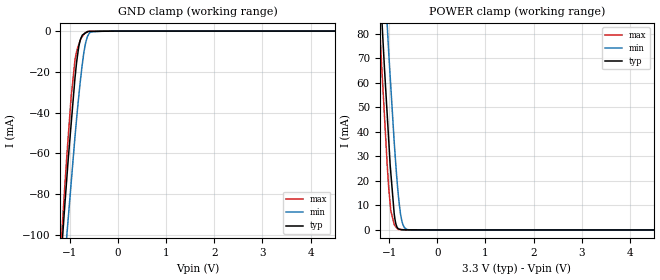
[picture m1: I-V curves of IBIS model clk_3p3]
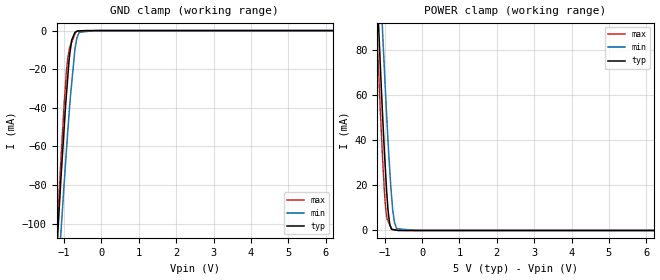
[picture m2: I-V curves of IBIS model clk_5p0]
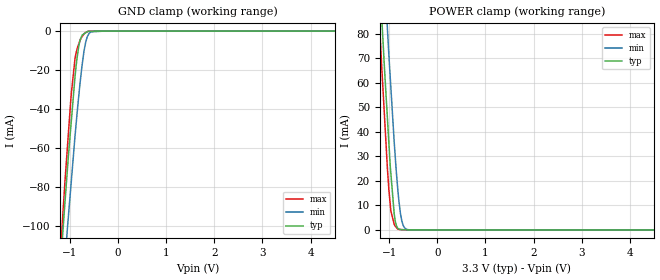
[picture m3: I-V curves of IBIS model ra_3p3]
|Texas Instruments Incorporated
| 10-Bit, 6 MSPS Simultaneous Sampling Quad Ch. ADC; Includes
| Parallel DSP/uP I/F & Ch. Auto-Scan
| Marketing part#   Digital Voltage Range   Package-type   #pins
| THS1007CDA   3.0V - 5.25V   TSSOP   32
| THS1007CDAG4   3.0V - 5.25V   TSSOP   32
| THS1007IDA   3.0V - 5.25V   TSSOP   32
| THS1007IDAG4   3.0V - 5.25V   TSSOP   32
[IBIS Ver]   3.2
[File name]   ths1007.ibs
[File Rev]   1.0
[Date]   2/6/2012
[Source]
| Texas Instruments Incorporated.
| Analog-eLab Design Center, HPA
| 12500 TI Blvd
| Dallas, TX -75243
| e-mail: elab_scm_ibis@list.ti.com
[Notes]   Revision History:
| Rev 1.0: 2/6/2012
| - Initial version of the model
| - Model generated from simulations in TISPICE
| - Model matched to SPICE simulation
| - C_comp although listed in numerical order of value are
|   obtained from varying PVT conditions. For PVT conditions for
|   each specific value refer the buffer description under
|   respective [Model]. IBIS model user is responsible for using
|   appropriate C_comp to simulate for Signal Integrity.
| - Model names with a trailing _3p3 contains the model for
|   3.3V [3.0V and 3.6V]. Model names with a trailing _5 contains
|   the model for 5.0V [4.75V and 5.25V].
[Disclaimer]
| This model is designed as an aid for customers of Texas Instruments.
| TI and its licensors and suppliers make no warranties, either expressed
| or implied, with respect to this  model, including the warranties of
| merchantability or fitness for a particular purpose. The model is
| provided solely on an "as is" basis. The entire risk as to its quality
| and performance is with the customer.
[Copyright]
 (C) Copyright 2011 Texas Instruments Incorporated.All rights reserved.
|   THS1007
[Component]   THS1007
[Manufacturer]   TI
[Package]   |32 TSSOP   -  DA package
|   typ   min   max
R_pkg   0.21688   0.20471   0.23277
L_pkg   3.61046nH   2.91278nH   5.42826nH
C_pkg   0.75773pF   0.65107pF   0.89681pF
[Pin]  signal_name   model_name   R_pin   L_pin   C_pin
1   D0   DB   0.22929   5.28549nH  0.88624pF
2   D1   DB   0.22246   4.29270nH  0.83152pF
3   D2   DB   0.22651   3.66644nH  0.76928pF
4   D3   DB   0.22257   3.58421nH  0.76689pF
5   D4   DB   0.21415   3.33153nH  0.75682pF
6   D5   DB   0.21138   3.18341nH  0.69847pF
7   BVDD   POWER   0.20869   3.00691nH  0.67046pF
8   BGND   GND   0.20684   2.88218nH  0.64638pF
9   D6   DB   0.21012   2.91278nH  0.66907pF
10   D7   DB   0.21063   3.01523nH  0.66849pF
11   D8   DB   0.21173   3.17954nH  0.69753pF
12   D9   DB   0.21581   3.34791nH  0.75697pF
13   RA0   RA   0.22106   3.56104nH  0.76788pF
14   RA1   RA   0.22704   3.67335nH  0.76968pF
15   CONV_CLK   CLK   0.22316   4.30100nH  0.83396pF
16   SYNC   NC   0.22970   5.28441nH  0.88787pF
17   DGND   GND   0.22638   5.25813nH  0.88757pF
18   DVDD   POWER   0.22209   4.28801nH  0.83532pF
19   _RD   INPUT   0.21868   3.58798nH  0.77751pF
20   _WR(R/_W)   INPUT   0.21332   3.49520nH  0.76759pF
21   CS1   INPUT   0.20861   3.28192nH  0.75570pF
22   _CS0   INPUT   0.20829   3.15463nH  0.69695pF
23   AVDD   POWER   0.21042   3.02121nH  0.66643pF
24   AGND   GND   0.12020   2.56007nH  0.68936pF
25   REFM   TERM   0.21206   2.92172nH  0.65107pF
26   REFP   TERM   0.21183   3.02353nH  0.67528pF
27   REFOUT   TERM   0.21699   3.22154nH  0.70177pF
28   REFIN   TERM   0.20471   3.24666nH  0.74948pF
29   BINM   TERM   0.20573   3.42657nH  0.72224pF
30   BINP   TERM   0.22780   3.70372nH  0.80843pF
31   AINM   TERM   0.21532   4.43526nH  0.86760pF
32   AINP   TERM   0.23277   5.42826nH  0.89681pF
1000   thermal_pad   NC   0.00003   0.00172nH  3.26032pF
|   Model Selectors
[Model Selector] CLK
clk_3p3  3.3V digital input
clk_5p0  5.0V digital input
[Model Selector] RA
ra_3p3  3.3V digital input
ra_5p0  5.0V digital input
[Model Selector] INPUT
input_3p3   3.3V digital input
input_5p0   5.0V digital input
[Model Selector] DB
db_3p3  3.3V digital I/O
db_5p0  5.0V digital I/O
[Model Selector] TERM
term_3-3V  3.3V nominal termination
term_5-0V  5.0V nominal termination
[Model] term_3-3V
Model_type Terminator
C_comp   1.0e-20F  1.0e-20F  1.0e-20F
|   typ   min   max
[Voltage Range]   3.3V   3.0V   3.6V
[POWER Clamp Reference]   3.3V   3.0V   3.6V
[GND Clamp Reference]   0V   0V   0V
|Ambient Temperature   25   85   -40
|Junction Temperature
[Temperature Range]   27   125   -40
[Model] term_5-0V
Model_type Terminator
C_comp   1.0e-20F  1.0e-20F  1.0e-20F
|   typ   min   max
[Voltage Range]   5.0V   4.75V   5.25V
[POWER Clamp Reference]   5.0V   4.75V   5.25V
[GND Clamp Reference]   0V   0V   0V
|Ambient Temperature   25   85   -40
|Junction Temperature
[Temperature Range]   27   125   -40
| Models and submodels in the file (10): clk_3p3 (Input), clk_5p0 (Input), ra_3p3 (Input), ra_5p0 (Input), input_3p3 (Input), input_5p0 (Input), db_3p3 (I/O), db_5p0 (I/O), term_3-3V (Terminator), term_5-0V (Terminator)
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|   clk_3p3 Model
[Model]   clk_3p3
Model_type   Input
Vinl = 0.6
Vinh = 2
|   typ   min   max
|   (nom PVT)   (fast PVT)   (slow PVT)
C_comp   1.043e-12   1.039e-12   1.060e-12
| Where nom  PVT is Nominal Process, 3.3V, 27C
| Fast PVT is Strong Process,  3.6V, -40C
| Slow PVT is Weak Process,   3V, 125C
[Voltage Range]   3.3   3   3.6
|Ambient Temperature   25   85   -40
|Junction Temperature
[Temperature Range]   27   125   -40
[Power Clamp Reference]   3.3   3   3.6
[GND Clamp Reference]   0   0   0
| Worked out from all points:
|   GND clamp passes 1 mA (typ) near -0.68 V on its own axis
|   POWER clamp passes 1 mA (typ) near -0.83 V on its own axis
[GND Clamp]
|   Voltage   I(typ)   I(min)   I(max)
-3.3V     -935.6mA   -897.7mA   -995.1mA
-1.224V   -123.9mA   -149mA     -118.7mA
-1.112V   -86.46mA   -114.3mA   -77.2mA
-1.062V   -70.38mA   -98.66mA   -59.48mA
-979.2mV  -46.05mA   -75.05mA   -32.84mA
-896.4mV  -22.69mA   -51.46mA   -13.92mA
-821.7mV  -8.032mA   -32.63mA   -6.791mA
-785.4mV  -4.151mA   -24.23mA   -4.431mA
-711mV    -1.434mA   -10.23mA   -1.518mA
-630.3mV  -168.3uA   -2.292mA   -315.6uA
-285mV    -75.61uA   -318nA     -92.94nA
6.6V      0A         0A         0A
[POWER Clamp]
|   Voltage   I(typ)   I(min)   I(max)
-3.3V     973mA      989.7mA    973.5mA
-1.29V    137.6mA    174.8mA    119.1mA
-1.155V   86.25mA    123.8mA    66.08mA
-1.102V   67mA       105mA      47.51mA
-1.037V   45.16mA    81.65mA    24.67mA
-968.4mV  23.51mA    58.7mA     7.943mA
-897.6mV  6.664mA    36.03mA    2.294mA
-810mV    491.8uA    13.94mA    237.7uA
-765mV    191.6uA    6.477mA    184.1uA
-714mV    63.15uA    2.037mA    123.5uA
-591mV    52.22uA    69.36uA    15.7uA
6.6V      0A         0A         0A
|   clk_5p0 Model
[Model]   clk_5p0
Model_type   Input
Vinl = 0.6
Vinh = 2.6
|   typ   min   max
|   (nom PVT)   (fast PVT)   (slow PVT)
C_comp   9.560e-13   9.523e-13   9.597e-13
| Where nom  PVT is Nominal Process, 5V, 27C
| Fast PVT is Strong Process,  5.25V, -40C
| Slow PVT is Weak Process,   4.75V, 125C
[Voltage Range]   5   4.75   5.25
|Ambient Temperature   25   85   -40
|Junction Temperature
[Temperature Range]   27   125   -40
[Power Clamp Reference]   5   4.75   5.25
[GND Clamp Reference]   0   0   0
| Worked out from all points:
|   GND clamp passes 1 mA (typ) near -0.71 V on its own axis
|   POWER clamp passes 1 mA (typ) near -0.83 V on its own axis
[GND Clamp]
|   Voltage   I(typ)   I(min)   I(max)
-5V       -1.642A    -1.561A    -1.74A
-1.306V   -152.3mA   -174.9mA   -150.2mA
-1.08V    -75.96mA   -104.1mA   -65.81mA
-997.5mV  -50.97mA   -79.67mA   -38.34mA
-939.7mV  -34.28mA   -63.54mA   -22.29mA
-897.8mV  -23.78mA   -51.82mA   -14.12mA
-855mV    -13.59mA   -40.68mA   -9.358mA
-795mV    -4.964mA   -27.44mA   -6.112mA
-707.7mV  -970.8uA   -9.742mA   -1.797mA
-640mV    -213.3uA   -3.087mA   -237.7uA
-190mV    0A         -23.35nA   -70.56uA
10V       0A         0A         0A
[POWER Clamp]
|   Voltage   I(typ)   I(min)   I(max)
-5V       1.711A     1.714A     1.72A
-1.306V   144.9mA    181.1mA    127mA
-1.113V   72.14mA    109.1mA    52.07mA
-1.054V   50.94mA    87.81mA    31.8mA
-966mV    22.96mA    57.47mA    8.774mA
-910mV    9.161mA    39.94mA    4.269mA
-860mV    2.43mA     25.95mA    2.444mA
-803.3mV  525.6uA    13.03mA    372.2uA
-736.2mV  316.1uA    3.495mA    231.3uA
-679.3mV  137.9uA    817.9uA    111.4uA
-190mV    0A         0A         8.884uA
10V       0A         0A         0A
|   ra_3p3 Model
[Model]   ra_3p3
Model_type   Input
Vinl = 0.6
Vinh = 2
|   typ   min   max
|   (nom PVT)   (fast PVT)   (slow PVT)
C_comp   1.043e-12   1.039e-12   1.060e-12
| Where nom  PVT is Nominal Process, 3.3V, 27C
| Fast PVT is Strong Process,  3.6V, -40C
| Slow PVT is Weak Process,   3V, 125C
[Voltage Range]   3.3   3   3.6
|Ambient Temperature   25   85   -40
|Junction Temperature
[Temperature Range]   27   125   -40
[Power Clamp Reference]   3.3   3   3.6
[GND Clamp Reference]   0   0   0
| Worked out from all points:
|   GND clamp passes 1 mA (typ) near -0.68 V on its own axis
|   POWER clamp passes 1 mA (typ) near -0.83 V on its own axis
[GND Clamp]
|   Voltage   I(typ)   I(min)   I(max)
-3.3V     -976mA     -939.6mA   -1.034A
-1.221V   -128mA     -154.9mA   -121.8mA
-1.109V   -88.8mA    -118.6mA   -78.24mA
-1.059V   -72.24mA   -102.5mA   -60.95mA
-979.2mV  -47.7mA    -78.56mA   -33.41mA
-896.4mV  -23.31mA   -53.77mA   -13.94mA
-821.7mV  -8.114mA   -33.97mA   -6.791mA
-785.4mV  -4.164mA   -25.18mA   -4.431mA
-714mV    -1.471mA   -10.96mA   -1.615mA
-633.6mV  -182.5uA   -2.489mA   -195.1uA
-285mV    -13.98uA   -318nA     -92.94nA
6.6V      0A         0A         0A
[POWER Clamp]
|   Voltage   I(typ)   I(min)   I(max)
-3.3V     973mA      989.7mA    973.5mA
-1.29V    137.6mA    174.8mA    119.1mA
-1.155V   86.25mA    123.8mA    66.08mA
-1.102V   67mA       105mA      47.51mA
-1.037V   45.16mA    81.65mA    24.67mA
-968.4mV  23.51mA    58.7mA     7.943mA
-897.6mV  6.664mA    36.03mA    2.294mA
-810mV    491.8uA    13.94mA    237.7uA
-765mV    191.6uA    6.477mA    184.1uA
-714mV    63.15uA    2.037mA    123.5uA
-591mV    52.22uA    69.36uA    15.7uA
6.6V      0A         0A         0A
